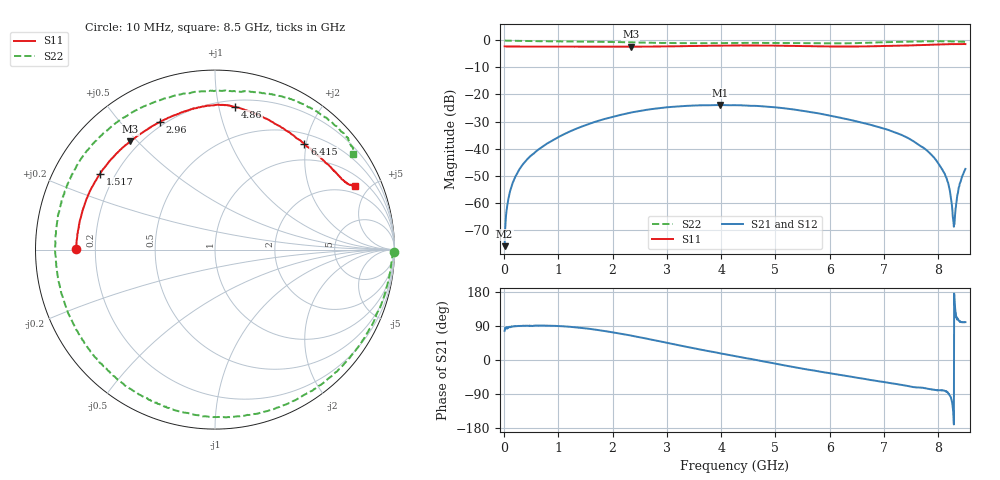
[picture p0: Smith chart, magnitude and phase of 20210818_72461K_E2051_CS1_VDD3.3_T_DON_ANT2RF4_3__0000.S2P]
!Agilent Technologies,E5071C,MY46417908,A.11.23
!Date: Wed Aug 18 14:32:40 2021
!Data & Calibration Information:
!Freq	S11:SOLT2(ON)	S21:SOLT2(ON)	S12:SOLT2(ON)	S22:SOLT2(ON)
!PortZ  Port1:50+j0  Port2:50+j0
!Above PortZ is port z conversion or system Z0 setting when saving the data.
!When reading, reference impedance value at option line is always used.
# Hz S dB R 50
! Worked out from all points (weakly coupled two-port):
!   1601 points, 10 MHz to 8.5 GHz, reference 50 ohm
!   highest |S21| = -23.91 dB at 3.979 GHz (marker M1); lowest = -76.1 dB at 10 MHz (marker M2)
!   lowest |S11| = -2.3 dB at 2.334 GHz (marker M3), VSWR 7.51, Z = 8.2 + j23.8 ohm
!   |S11| at or under -10 dB: nowhere
!   |S22| runs from -1.1 to 0.0 dB; largest |S21 - S12| = 0.00033
!   S11 on the Smith chart (normalised r, x): 10 MHz: 0.13, +0.00; 1.517 GHz: 0.14, +0.30; 2.96 GHz: 0.18, +0.64; 4.86 GHz: 0.25, +1.12; 6.415 GHz: 0.67, +1.97; 8.5 GHz: 1.52, +4.03
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1e7  -2.20 179.7  -76.13 76.9  -75.81 83.2  -0.01 -0.6
6.836875e7  -2.24 178.4  -60.06 86.1  -60.00 85.7  -0.11 -3.2
1.16125e8  -2.24 177.3  -55.43 86.6  -55.48 87.8  -0.13 -5.3
3.230688e8  -2.27 172.5  -46.49 90.1  -46.51 90.2  -0.19 -14.2
7.581812e8  -2.29 162.8  -38.62 90.9  -38.61 91.0  -0.30 -32.4
1.426769e9  -2.30 148.5  -31.90 84.6  -31.92 84.5  -0.45 -60.9
1.516975e9  -2.30 146.5  -31.25 83.2  -31.26 83.1  -0.45 -64.8
2.334138e9  -2.33 128.0  -26.71 64.6  -26.71 64.5  -0.70 -103.1
2.843538e9  -2.24 115.9  -25.10 50.0  -25.11 50.0  -0.89 -129.1
2.960275e9  -2.21 113.2  -24.83 46.7  -24.81 46.7  -0.92 -135.2
3.480288e9  -2.06 102.5  -24.11 31.6  -24.11 31.6  -1.02 -162.2
3.979075e9  -1.93 94.1  -23.91 17.7  -23.92 17.8  -0.99 173.3
4.255e9  -1.88 90.0  -23.97 10.5  -23.98 10.6  -0.94 160.5
4.859912e9  -1.90 82.1  -24.53 -5.8  -24.54 -5.8  -0.93 135.0
5.671769e9  -2.13 67.6  -26.61 -27.0  -26.60 -27.0  -1.04 104.3
6.414644e9  -2.25 49.8  -29.55 -44.6  -29.55 -44.7  -1.01 83.0
7.088538e9  -2.02 35.2  -33.20 -60.5  -33.24 -60.6  -0.61 65.8
7.932231e9  -1.55 25.5  -43.56 -78.7  -43.63 -79.0  -0.31 44.8
8.1604e9  -1.40 25.0  -51.38 -83.6  -51.35 -85.1  -0.29 39.9
8.28775e9  -1.37 24.9  -68.94 -170.1  -68.81 -169.0  -0.40 38.0
8.404488e9  -1.36 24.7  -52.59 100.4  -52.57 102.0  -0.45 36.0
8.5e9  -1.36 24.7  -47.55 99.9  -47.53 99.5  -0.56 34.8
